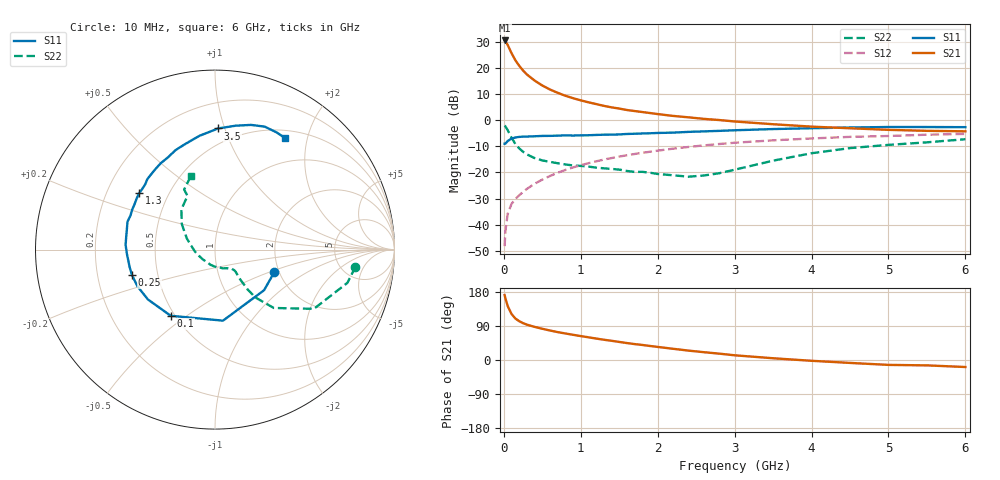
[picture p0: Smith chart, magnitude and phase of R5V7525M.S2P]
! SIEMENS Small Signal Semiconductors
! BFR183
! Si NPN RF Bipolar Junction Transistor in SOT23
! VCE = 0.75 V  IC = 25 mA
! Common Emitter S-Parameters:  May  1996
# GHz  S  MA  R  50
!  f  S11  S21  S12  S22
! GHz  MAG  ANG  MAG  ANG  MAG  ANG  MAG  ANG
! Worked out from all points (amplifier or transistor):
!   36 points, 10 MHz to 6 GHz, reference 50 ohm
!   highest |S21| = 30.5 dB at 10 MHz (marker M1)
!   |S21| within 3 dB of that: start of sweep to 70.45 MHz
!   unconditionally stable (mu >= 1): start of sweep to 14.35 MHz; 232.9 MHz to end of sweep
!   at 250 MHz: K = 1.03, MAG = 22.2 dB, |S12| = -27.4 dB
!   at 1.4 GHz: K = 1.19, MAG = 7.0 dB, |S12| = -14.5 dB
!   at 6 GHz: K = 1.04, MAG = -0.8 dB, |S12| = -5.3 dB
!   S11 on the Smith chart (normalised r, x): 10 MHz: 1.89, -0.54; 100 MHz: 0.48, -0.44; 250 MHz: 0.36, -0.13; 1.3 GHz: 0.34, +0.30; 3.5 GHz: 0.38, +0.95; 6 GHz: 0.61, +1.64
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0.01  0.3537 -20.6  33.32 171.3  0.0039 80.5  0.788 -7.0
0.02  0.3549 -39.6  32.3 162.9  0.0075 74.7  0.7605 -14.1
0.05  0.3984 -83.6  27.33 142.3  0.0162 66.6  0.6426 -30.9
0.1  0.4437 -123.8  19.06 121.4  0.0251 60.0  0.4616 -44.8
0.15  0.4658 -143.4  13.93 109.5  0.0311 59.3  0.3497 -49.8
0.2  0.4779 -154.6  10.93 102.4  0.0366 60.9  0.2879 -50.7
0.25  0.4836 -162.8  8.863 97.2  0.0425 62.6  0.2482 -50.3
0.3  0.4855 -168.3  7.446 93.3  0.0485 64.6  0.221 -49.9
0.4  0.4913 -177.2  5.7 87.4  0.0608 66.4  0.1883 -48.4
0.5  0.4988 177.0  4.591 82.4  0.073 67.8  0.1699 -47.1
0.6  0.5001 171.3  3.845 77.8  0.0856 67.9  0.1592 -46.9
0.7  0.5047 166.4  3.327 73.6  0.0986 67.6  0.1501 -47.8
0.8  0.5117 162.3  2.923 70.0  0.1116 66.9  0.1421 -48.9
1.1  0.5144 150.8  2.191 59.9  0.1502 64.6  0.1295 -54.8
1.3  0.5264 143.3  1.874 53.5  0.1762 62.0  0.12 -59.7
1.6  0.5441 133.9  1.561 44.7  0.2133 58.1  0.1068 -72.1
2.2  0.5768 117.1  1.204 29.6  0.2849 49.5  0.0882 -107.0
2.6  0.6093 106.4  1.057 20.6  0.3288 43.4  0.0874 -141.8
3.5  0.6753 88.5  0.835 4.6  0.4111 29.3  0.168 158.7
4.5  0.7231 73.9  0.699 -7.7  0.4787 15.2  0.2918 130.0
5.5  0.7378 62.3  0.624 -14.2  0.5268 3.6  0.3763 117.2
6  0.734 57.8  0.611 -18.5  0.5458 -3.6  0.4319 108.0
